FUNCTION_BLOCK FB_FileCopy
VAR_INPUT
	sSrcNetId			: T_AmsNetId;	(* TwinCAT network address of the source file *)
	sSrcPathName		: T_MaxString;	(* Source file path and name *)
	sDestNetId			: T_AmsNetId;	(* TwinCAT network address of the destination file *)
	sDestPathName		: T_MaxString;  (* Destination file path and name *)
	bExecute			: BOOL;			(* Rising edge start fb execution *)
	tTimeOut			: TIME := DEFAULT_ADS_TIMEOUT;(* Max. ADS timeout time *)
END_VAR
VAR_OUTPUT
	bBusy				:BOOL;(* TRUE => File copy execution in progress, FALSE => File copy execution idle *)
	bError				:BOOL;(* TRUE => Error, FALSE => No error *)
	nErrId				:UDINT;(* Error code *)
END_VAR
VAR
	fbFileOpen			:FB_FileOpen;
	fbFileClose			:FB_FileClose;
	fbFileRead			:FB_FileRead;
	fbFileWrite			:FB_FileWrite;

	hSrcFile			:UINT	:= 0;(* File handle of the source file *)
	hDestFile			:UINT	:= 0;(* File handle of the destination file *)

	Step				:DWORD;
	RisingEdge			:R_TRIG;

	buffRead			:ARRAY[1..1000] OF BYTE;(* Buffer *)
	cbReadLength		:UDINT := 0;
END_VAR

RisingEdge(CLK:=bExecute);

CASE Step OF
	0:	(* Idle state *)
		IF RisingEdge.Q THEN
			bBusy := TRUE;
			bError:= FALSE;
			nErrId:=0;
			Step := 1;
			cbReadLength:=0;
			hSrcFile:=0;
			hDestFile:=0;
		END_IF

	1:	(* Open source file *)
		fbFileOpen( bExecute := FALSE );
		fbFileOpen( sNetId := sSrcNetId, sPathName := sSrcPathName,
					nMode := FOPEN_MODEREAD OR FOPEN_MODEBINARY,
					ePath := PATH_GENERIC, tTimeout := tTimeOut, bExecute := TRUE );
		Step := Step + 1;
	2:
		fbFileOpen( bExecute := FALSE );
		IF NOT fbFileOpen.bBusy THEN
			IF fbFileOpen.bError THEN
				nErrId := fbFileOpen.nErrId;
				bError := TRUE;
				Step := 50;
			ELSE
				hSrcFile := fbFileOpen.hFile;
				Step := Step + 1;
			END_IF
		END_IF

	3:	(* Open destination file *)
		fbFileOpen( bExecute := FALSE );
		fbFileOpen( sNetId := sDestNetId, sPathName := sDestPathName,
					nMode := FOPEN_MODEWRITE OR FOPEN_MODEBINARY,
					ePath := PATH_GENERIC, tTimeout := tTimeOut, bExecute := TRUE );
		Step := Step+1;
	4:
		fbFileOpen( bExecute := FALSE );
		IF NOT fbFileOpen.bBusy THEN
			IF fbFileOpen.bError THEN
				nErrId := fbFileOpen.nErrId;
				bError := TRUE;
				Step := 50;
			ELSE
				hDestFile := fbFileOpen.hFile;
				Step := Step + 1;
			END_IF
		END_IF

	5:	(* Read data from source file *)
		cbReadLength := 0;
		fbFileRead( bExecute:= FALSE );
		fbFileRead( sNetId:=sSrcNetId, hFile:=hSrcFile,
					pReadBuff:= ADR(buffRead), cbReadLen:= SIZEOF(buffRead),
					bExecute:=TRUE, tTimeout:=tTimeOut );
		Step := Step + 1;
	6:
		fbFileRead( bExecute:= FALSE );
		IF NOT fbFileRead.bBusy THEN
			IF fbFileRead.bError THEN
				nErrId := fbFileRead.nErrId;
				bError := TRUE;
				Step := 50;
			ELSE
				cbReadLength := fbFileRead.cbRead;
				Step := Step + 1;
			END_IF
		END_IF

	7:	(* Write data to destination file *)
		fbFileWrite( bExecute := FALSE );
		fbFileWrite( sNetId:=sDestNetId, hFile:=hDestFile,
					pWriteBuff:= ADR(buffRead), cbWriteLen:= cbReadLength,
					bExecute:=TRUE, tTimeout:=tTimeOut );
		Step := Step + 1;
	8:
		fbFileWrite( bExecute := FALSE );
		IF NOT fbFileWrite.bBusy THEN
			IF fbFileWrite.bError THEN
				nErrId := fbFileWrite.nErrId;
				bError := TRUE;
				Step := 50;
			ELSE
				IF fbFileRead.bEOF THEN (* Check if the EOF flag ist set *)
					Step := 50;	(* Cleanup: close the destination and source files *)
				ELSE
					Step := 5; (* Repeat reading/writing *)
				END_IF
			END_IF
		END_IF

	30:	(* Close the destination file *)
		fbFileClose( bExecute := FALSE );
		fbFileClose( sNetId:=sDestNetId, hFile:=hDestFile, bExecute:=TRUE, tTimeout:=tTimeOut );
		Step := Step + 1;
	31:
		fbFileClose( bExecute := FALSE );
		IF NOT fbFileClose.bBusy THEN
			IF fbFileClose.bError THEN
				nErrId := fbFileClose.nErrId;
				bError := TRUE;
			END_IF
			Step := 50;
			hDestFile := 0;
		END_IF

	40: (* Close source file *)
		fbFileClose( bExecute := FALSE );
		fbFileClose( sNetId:=sSrcNetId, hFile:=hSrcFile, bExecute:=TRUE, tTimeout:=tTimeOut );
		Step := Step + 1;
	41:
		fbFileClose( bExecute := FALSE );
		IF NOT fbFileClose.bBusy THEN
			IF fbFileClose.bError THEN
				nErrId := fbFileClose.nErrId;
				bError := TRUE;
			END_IF
			Step := 50;
			hSrcFile := 0;
		END_IF

	50: (* Error or ready => Cleanup *)
		IF ( hDestFile <> 0 ) THEN
			Step := 30; (* Close the destination file*)
		ELSIF (hSrcFile <> 0 ) THEN
			Step := 40; (* Close the source file *)
		ELSE
			Step := 0;	(* Ready *)
			bBusy := FALSE;
		END_IF

END_CASE

END_FUNCTION_BLOCK
